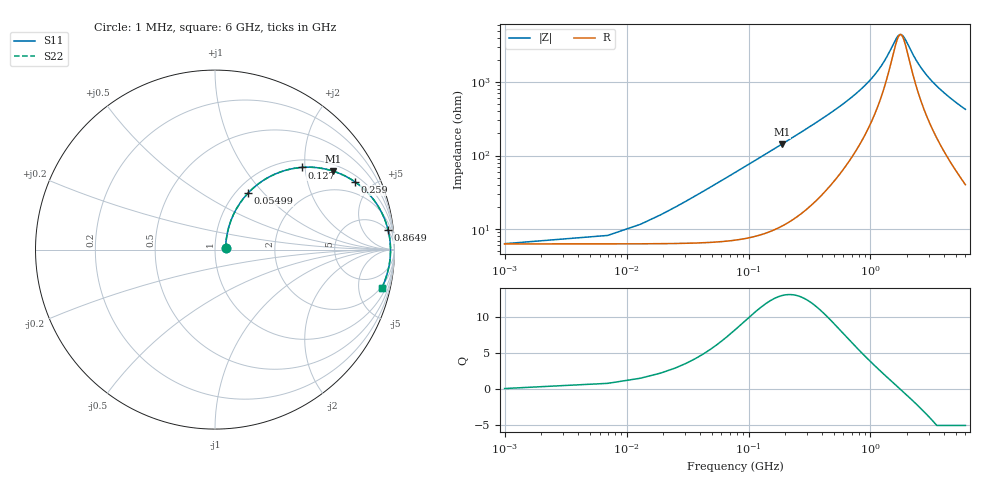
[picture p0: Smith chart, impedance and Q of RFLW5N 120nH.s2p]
!Vishay Electro-Films
!RFLW5N1200A - 120 nH Spiral Inductor on Quartz
!Measured in series configuration
!May 2011
# GHz S MA R 50
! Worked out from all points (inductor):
!   1001 points, 1 MHz to 6 GHz, reference 50 ohm
!   read as one part in series: L = 120 nH near 31 MHz
!   highest Q = 13 at 187 MHz (marker M1), where L = 121 nH
!   self-resonance near 1.762 GHz
!   S11 on the Smith chart (normalised r, x): 1 MHz: 1.13, +0.02; 54.99 MHz: 1.13, +0.83; 127 MHz: 1.17, +1.92; 259 MHz: 1.31, +3.97; 864.9 MHz: 4, +16; 6 GHz: 1.80, -8.46
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0.001  0.05961 6.4  0.9408 -0.4  0.9408 -0.4  0.05961 6.4
0.018997  0.1457 58.4  0.932 -7.7  0.932 -7.7  0.1457 58.4
0.042993  0.2964 61.7  0.8982 -16.9  0.8982 -16.9  0.2964 61.7
0.054991  0.3663 59.6  0.8739 -21.2  0.8739 -21.2  0.3663 59.6
0.084986  0.5159 52.7  0.8007 -30.8  0.8007 -30.8  0.5159 52.7
0.126979  0.6652 43.5  0.6908 -41.5  0.6908 -41.5  0.6652 43.5
0.186969  0.7904 33.6  0.5549 -52.0  0.5549 -52.0  0.7904 33.6
0.258957  0.8673 25.7  0.4354 -59.8  0.4354 -59.8  0.8673 25.7
0.348942  0.9141 19.5  0.3348 -65.6  0.3348 -65.6  0.9141 19.5
0.462923  0.9421 14.5  0.2525 -69.6  0.2525 -69.6  0.9421 14.5
0.864856  0.9706 6.5  0.1153 -72.0  0.1153 -72.0  0.9706 6.5
1.00283  0.9735 5.0  0.08994 -70.4  0.08994 -70.4  0.9735 5.0
1.58474  0.9777 0.9  0.02711 -34.3  0.02711 -34.3  0.9777 0.9
1.68072  0.9779 0.4  0.02318 -17.0  0.02318 -17.0  0.9779 0.4
1.8187  0.9779 -0.3  0.02255 11.7  0.02255 11.7  0.9779 -0.3
2.00467  0.9778 -1.1  0.02911 39.8  0.02911 39.8  0.9778 -1.1
2.22663  0.9775 -2.0  0.04111 55.8  0.04111 55.8  0.9775 -2.0
2.44859  0.9769 -2.8  0.05393 63.2  0.05393 63.2  0.9769 -2.8
3.0005  0.9749 -4.7  0.08473 70.4  0.08473 70.4  0.9749 -4.7
4.00233  0.9694 -7.7  0.1354 73.1  0.1354 73.1  0.9694 -7.7
5.00417  0.9622 -10.4  0.1815 72.8  0.1815 72.8  0.9622 -10.4
6  0.9535 -12.9  0.2244 71.7  0.2244 71.7  0.9535 -12.9
